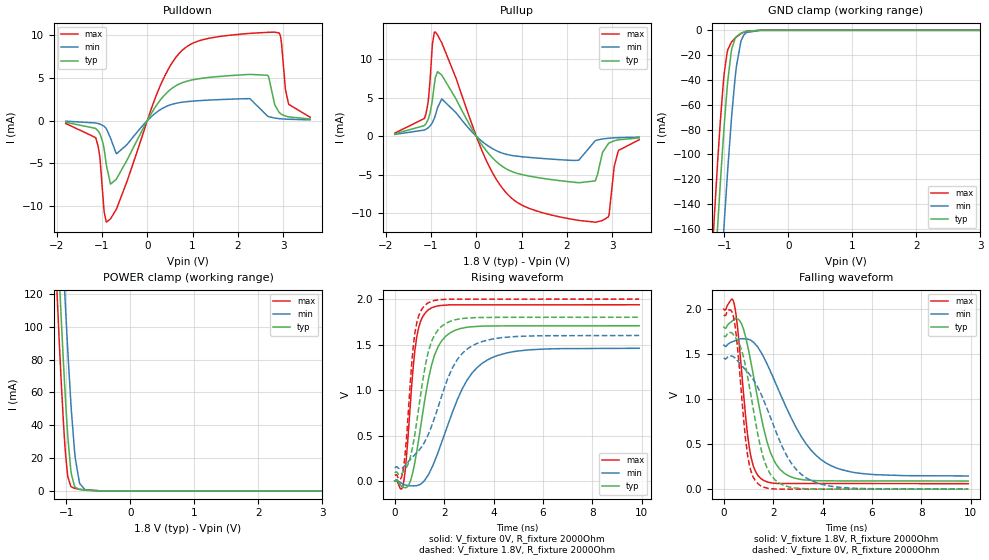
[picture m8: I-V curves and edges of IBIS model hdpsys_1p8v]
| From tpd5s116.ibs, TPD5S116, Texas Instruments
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[Model]   hdpsys_1p8v
Model_type   3-state
Polarity   Non-Inverting
Vmeas = 0.9
Vref = 1.8
Cref = 15pF
Rref = 2000
|   typ   min   max
|   (nom PVT)   (slow PVT)   (fast PVT)
C_comp   1.1241p   1.0342p   1.3025p
|C_comp (High state)   1.1241p   1.0342p   1.3025p
|C_comp (Low state)   1.0197p   0.970p   1.0858p
| Where nom  PVT is Nominal Process, 1.8V, 27C
|   Fast PVT is Strong Process,  2.0V, -40C
|   Slow PVT is Weak Process,   1.6V, 125C
[Voltage Range]   1.8   1.6   2
[Temperature Range]   27   125   -40
[Pullup Reference]   1.8   1.6   2
[Pulldown Reference]   -0   -0   -0
[Power Clamp Reference]   1.8   1.6   2
[GND Clamp Reference]   -0   -0   -0
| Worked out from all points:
|   slope of the pulldown table from 0 to 0.27 V, typ, clamps not added: 118 ohm
|   slope of the pullup table from 0 to 0.27 V, typ, clamps not added: 121 ohm
|   GND clamp passes 1 mA (typ) near -0.67 V on its own axis
|   POWER clamp passes 1 mA (typ) near -0.80 V on its own axis
|   falling waveform, V_fixture 1.8V, R_fixture 2000Ohm: 20-80 % time 797ps typ, 1.63ns min, 417ps max; typ from 1.8 V to 0.091 V
|   rising waveform, V_fixture 0V, R_fixture 2000Ohm: 20-80 % time 688ps typ, 1.36ns min, 362ps max; typ from 0 V to 1.71 V
|   rising waveform, V_fixture 1.8V, R_fixture 2000Ohm: 20-80 % time 639ps typ, 1.25ns min, 341ps max; typ from 0.091 V to 1.8 V
|   falling waveform, V_fixture 0V, R_fixture 2000Ohm: 20-80 % time 730ps typ, 1.42ns min, 395ps max; typ from 1.71 V to 0 V
[Pulldown]
|   Voltage   I(typ)   I(min)   I(max)
-1.8V     -200.2uA   -73.09uA   -339uA
-1.141V   -912.6uA   -278.8uA   -1.984mA
-1.049V   -1.511mA   -403uA     -4.187mA
-903.6mV  -5.202mA   -950.3uA   -11.86mA
-676.8mV  -6.782mA   -3.864mA   -10.27mA
333mV     2.695mA    1.417mA    4.629mA
981mV     4.732mA    2.26mA     8.968mA
2.266V    5.387mA    2.559mA    10.18mA
2.655V    5.291mA    508.6uA    10.3mA
2.909V    953.2uA    226.8uA    10.22mA
3.119V    426.8uA    152.3uA    1.9mA
3.595V    182.8uA    86.38uA    385uA
[GND Clamp]
|   Voltage   I(typ)   I(min)   I(max)
-1.8V     -807.2mA   -889.1mA   -756.3mA
-1.195V   -236.5mA   -321.3mA   -182.9mA
-1.103V   -156.4mA   -240.1mA   -104.5mA
-1.06V    -120.7mA   -203.1mA   -71.14mA
-1.006V   -79.23mA   -158.3mA   -36.67mA
-957.6mV  -46.93mA   -120mA     -18.13mA
-892.8mV  -17.42mA   -73.65mA   -9.707mA
-811.8mV  -5.048mA   -29.01mA   -5.339mA
-741.6mV  -2.35mA    -8.858mA   -2.701mA
-655.2mV  -807.9uA   -1.783mA   -788uA
-450mV    -15.5uA    -52.27uA   -6.571uA
3.595V    0A         0A         0A
[Pullup]
|   Voltage   I(typ)   I(min)   I(max)
-1.8V     326.7uA    247.6uA    417.3uA
-1.147V   1.391mA    814.1uA    2.307mA
-903.6mV  7.646mA    2.736mA    13.54mA
-763.2mV  7.959mA    4.859mA    12.15mA
279mV     -2.293mA   -1.324mA   -3.858mA
986.4mV   -4.945mA   -2.64mA    -8.879mA
2.25V     -6.024mA   -3.097mA   -10.91mA
2.623V    -5.794mA   -581uA     -11.16mA
2.785V    -2.097mA   -343.8uA   -10.94mA
2.93V     -877.1uA   -247.7uA   -10.14mA
3.136V    -450.9uA   -176.3uA   -1.849mA
3.595V    -209.7uA   -106.3uA   -437.8uA
[POWER Clamp]
|   Voltage   I(typ)   I(min)   I(max)
-1.8V     773.1mA    829.3mA    737.4mA
-1.211V   217.6mA    278.5mA    177.8mA
-1.109V   128.8mA    189.3mA    89.43mA
-1.087V   111.1mA    171.2mA    72.27mA
-1.049V   81.52mA    140.3mA    44.65mA
-1.022V   61.86mA    119mA      27.87mA
-973.8mV  31.45mA    83.01mA    8.282mA
-919.8mV  9.913mA    48.1mA     2.424mA
-860.4mV  2.216mA    19.89mA    1.488mA
-795.6mV  848.7uA    5.082mA    1.054mA
-709.2mV  419uA      759uA      591.6uA
3.595V    0A         0A         0A
[Ramp]
R_load = 2000
|   typ   min   max
dV/dt_r   1.02384/6.88093e-10   0.875403/1.35755e-09   1.16234/3.62192e-10
dV/dt_f   1.02562/7.96714e-10   0.8719/1.63363e-09   1.16319/4.17467e-10
[Falling Waveform]
V_fixture = 1.8V
V_fixture_min = 1.6V
V_fixture_max = 2V
R_fixture = 2000Ohm
C_fixture = 0F
|   Time   V(typ)   V(min)   V(max)
0s        1.8V       1.6V       2V
418ps     1.884V     1.645V     2.063V
719.1ps   1.836V     1.671V     1.319V
1.032ns   1.503V     1.661V     462.7mV
1.488ns   839.1mV    1.53V      120.6mV
1.894ns   405mV      1.306V     72.25mV
2.255ns   225.6mV    1.079V     62.91mV
3.132ns   108.1mV    586.8mV    62.73mV
4.132ns   92.95mV    292.2mV    62.53mV
9.9ns     90.64mV    146.8mV    61.36mV
[Rising Waveform]
V_fixture = 0V
V_fixture_min = 0V
V_fixture_max = 0V
R_fixture = 2000Ohm
C_fixture = 0F
|   Time   V(typ)   V(min)   V(max)
0s        3.976nV    202.3nV    1.21nV
349.3ps   -69.27mV   -34.21mV   -28.61mV
468ps     -70.35mV   -46.7mV    246.9mV
639.7ps   4.154mV    -52.16mV   877.7mV
885.5ps   316.3mV    -50.41mV   1.577V
1.377ns   1.137V     77.11mV    1.885V
2.074ns   1.594V     558.5mV    1.934V
2.932ns   1.69V      1.111V     1.936V
3.732ns   1.704V     1.328V     1.936V
9.9ns     1.706V     1.459V     1.937V
[Rising Waveform]
V_fixture = 1.8V
V_fixture_min = 1.6V
V_fixture_max = 2V
R_fixture = 2000Ohm
C_fixture = 0F
|   Time   V(typ)   V(min)   V(max)
0s        90.52mV    146.3mV    61.35mV
325.4ps   94.1mV     146.9mV    97.33mV
418ps     127.4mV    173mV      294.2mV
579.3ps   216.3mV    222.1mV    881.8mV
812ps     512.6mV    289mV      1.621V
1.287ns   1.333V     472.2mV    1.946V
1.599ns   1.599V     686.4mV    1.984V
2.332ns   1.763V     1.243V     1.999V
3.332ns   1.797V     1.512V     1.999V
9.9ns     1.8V       1.6V       2V
[Falling Waveform]
|Gnd
V_fixture = 0V
V_fixture_min = 0V
V_fixture_max = 0V
R_fixture = 2000Ohm
C_fixture = 0F
|   Time   V(typ)   V(min)   V(max)
0s        1.707V     1.459V     1.937V
379.2ps   1.719V     1.473V     1.93V
518ps     1.666V     1.439V     1.674V
959ps     1.258V     1.302V     387.2mV
1.196ns   887.9mV    1.218V     131.1mV
1.488ns   467.5mV    1.067V     39.08mV
2.074ns   103.1mV    666.1mV    1.783mV
2.732ns   20.21mV    289.1mV    286.8uV
3.532ns   2.535mV    96.07mV    255.3uV
9.9ns     102.3uV    311.6uV    4.338uV
